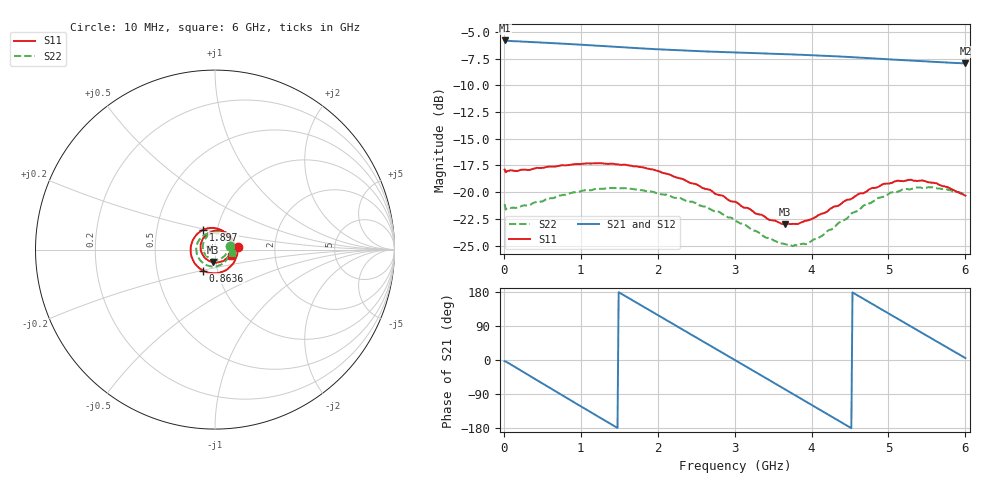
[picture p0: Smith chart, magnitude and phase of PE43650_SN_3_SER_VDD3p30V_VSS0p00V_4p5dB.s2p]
!Keysight Technologies,N5245B,MY57181451,A.13.50.07
!Date: Tuesday, May 07, 2019 07:59:53
!Correction: S11(Full 2 Port(1,2))
!S21(Full 2 Port(1,2))
!S12(Full 2 Port(1,2))
!S22(Full 2 Port(1,2))
!S2P File: Measurements: S11, S21, S12, S22:
# Hz S  dB  R 50
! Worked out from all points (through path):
!   401 points, 10 MHz to 6 GHz, reference 50 ohm
!   highest |S21| = -5.81 dB at 10 MHz (marker M1); lowest = -8.0 dB at 6 GHz (marker M2)
!   group delay of S21, straight-line fit = 330 ps
!   lowest |S11| = -23.0 dB at 3.649 GHz (marker M3), VSWR 1.15, Z = 48.2 - j6.75 ohm
!   |S11| at or under -10 dB: start of sweep to end of sweep
!   |S22| runs from -25.1 to -19.5 dB; largest |S21 - S12| = 0.0037
!   S11 on the Smith chart (normalised r, x): 10 MHz: 1.29, +0.04; 863.6 MHz: 0.85, -0.20; 1.897 GHz: 0.86, +0.19; 6 GHz: 1.19, -0.09
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1e7  -17.89 7.3  -5.81 -3.3  -5.87 -3.3  -21.12 13.3
2.34625e8  -17.90 -34.3  -5.91 -29.4  -5.96 -29.4  -21.28 -35.0
4.892e8  -17.73 -69.8  -6.00 -60.4  -6.06 -60.4  -20.86 -71.3
8.63575e8  -17.45 -119.5  -6.15 -105.7  -6.20 -105.7  -20.09 -120.4
1.013325e9  -17.37 -138.3  -6.22 -123.7  -6.27 -123.7  -19.88 -138.4
1.4476e9  -17.38 170.7  -6.40 -175.7  -6.46 -175.7  -19.62 173.4
1.89685e9  -17.83 120.9  -6.59 130.8  -6.65 130.9  -19.95 127.4
2.01665e9  -18.06 108.1  -6.64 116.6  -6.69 116.7  -20.13 115.7
2.241275e9  -18.63 83.8  -6.72 90.1  -6.78 90.1  -20.53 93.3
2.4659e9  -19.20 58.8  -6.79 63.5  -6.85 63.5  -20.94 70.9
2.750425e9  -20.17 26.9  -6.87 29.9  -6.92 30.0  -21.79 40.7
3.005e9  -20.89 -5.2  -6.93 -0.2  -6.99 -0.2  -22.59 11.8
3.3045e9  -22.06 -46.7  -7.00 -35.8  -7.05 -35.7  -23.75 -28.4
3.648925e9  -22.99 -100.7  -7.09 -76.6  -7.14 -76.6  -24.84 -82.0
4.008325e9  -22.49 -159.9  -7.19 -119.3  -7.24 -119.3  -24.52 -143.7
4.2629e9  -21.49 161.8  -7.28 -149.6  -7.33 -149.6  -23.47 176.0
4.5025e9  -20.68 129.0  -7.37 -178.1  -7.42 -178.0  -22.13 141.7
4.7421e9  -19.78 98.9  -7.47 153.4  -7.52 153.6  -21.07 112.6
5.01165e9  -19.19 68.8  -7.58 121.6  -7.63 121.7  -20.11 81.6
5.4609e9  -18.94 23.3  -7.75 68.6  -7.80 68.7  -19.61 36.8
5.745425e9  -19.49 -2.0  -7.87 35.0  -7.92 35.1  -19.71 11.0
6e9  -20.32 -22.2  -7.96 5.1  -8.01 5.2  -20.27 -10.1
